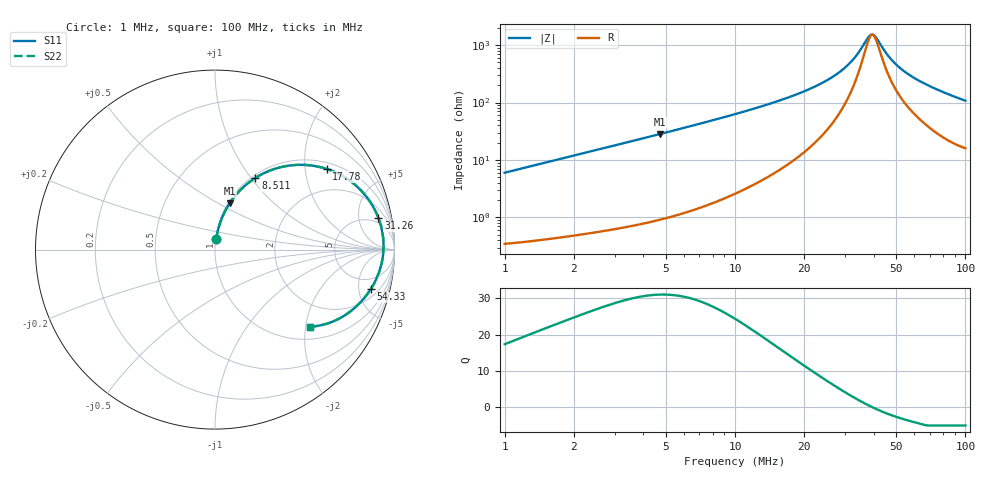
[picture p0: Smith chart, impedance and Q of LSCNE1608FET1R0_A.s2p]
! LSCNE1608FET1R0_A  S-PARAMETER MODEL  ( Standard Model )
! Model Generated by TAIYO YUDEN Corporation (http://www.ty-top.com)
! Version 1.0
! TAIYO YUDEN Control No. 160926
! Copyright(c) 2016 TAIYO YUDEN CO.,LTD. All Rights Reserved.
! Product Description (link to TY-COMPAS)
! https://ds.yuden.co.jp/TYCOMPAS/or/detail?pn=LSCNE1608FET1R0MA&u=M
! Products Name : Inductors
! Characteristics :
!  Inductance : 1.0 [uH] , SRF(min) : - [Hz] , DC Resistance(max) : 340 [mOhm]
!  Rated Current : Saturation  1.4 [A] (dL = 30 [%]), Temp Rise  0.8 [A] (dT = 40 [degC])
!  Case Size : 1.6 x 0.8 / 0.063 x 0.031 [mm/inch] , Thickness : 0.65 / 0.026 [mm/inch]
!  (Conditions: Temperature = 25 [degC] , DC Bias Current = 0 [A])
! External Node Assignments :
!  1  o---GGG---o  2
! GND o---------o GND
! Frequency Range : 1MHz  -  100MHz  [ 402 STEP ]
# MHz S RI R 50
! Freq[MHz].  S11 Real  S11 Imag  S21 Real  S21 Imag  S12 Real  S12 Imag  S22 Real  S22 Imag
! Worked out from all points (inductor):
!   401 points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, 1 MHz to 100 MHz, reference 50 ohm
!   read as one part in series: L = 952 nH near 1.023 MHz
!   highest Q = 31 at 4.732 MHz (marker M1), where L = 953 nH
!   self-resonance near 39.5 MHz
!   S11 on the Smith chart (normalised r, x): 1 MHz: 1.01, +0.12; 8.511 MHz: 1.04, +1.05; 17.78 MHz: 1.19, +2.61; 31.26 MHz: 3.61, +9.06; 54.33 MHz: 3.00, -6.67; 100 MHz: 1.32, -2.13
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1  0.007 0.0594  0.993 -0.0594  0.993 -0.0594  0.007 0.0594
1.62181  0.0135 0.0952  0.9865 -0.0952  0.9865 -0.0952  0.0135 0.0952
2.42661  0.0256 0.1401  0.9744 -0.1401  0.9744 -0.1401  0.0256 0.1401
3.467369  0.047 0.1956  0.953 -0.1956  0.953 -0.1956  0.047 0.1956
4.731513  0.0814 0.2578  0.9186 -0.2578  0.9186 -0.2578  0.0814 0.2578
6.456542  0.1407 0.3314  0.8593 -0.3314  0.8593 -0.3314  0.1407 0.3314
8.51138  0.2247 0.3992  0.7753 -0.3992  0.7753 -0.3992  0.2247 0.3992
12.73503  0.4148 0.4683  0.5852 -0.4683  0.5852 -0.4683  0.4148 0.4683
17.57924  0.6144 0.4519  0.3856 -0.4519  0.3856 -0.4519  0.6144 0.4519
17.78279  0.6218 0.4496  0.3782 -0.4496  0.3782 -0.4496  0.6218 0.4496
24.2661  0.8083 0.335  0.1917 -0.335  0.1917 -0.335  0.8083 0.335
31.26079  0.9108 0.1754  0.0892 -0.1754  0.0892 -0.1754  0.9108 0.1754
34.27678  0.9303 0.1077  0.0697 -0.1077  0.0697 -0.1077  0.9303 0.1077
38.01894  0.939 0.029  0.061 -0.029  0.061 -0.029  0.939 0.029
39.81072  0.9383 -0.00594  0.0617 0.00594  0.0617 0.00594  0.9383 -0.00594
41.20975  0.9359 -0.032  0.0641 0.032  0.0641 0.032  0.9359 -0.032
46.2381  0.9174 -0.1157  0.0826 0.1157  0.0826 0.1157  0.9174 -0.1157
50.69907  0.8919 -0.1777  0.1081 0.1777  0.1081 0.1777  0.8919 -0.1777
54.32503  0.8677 -0.2204  0.1323 0.2204  0.1323 0.2204  0.8677 -0.2204
67.6083  0.7682 -0.3333  0.2318 0.3333  0.2318 0.3333  0.7682 -0.3333
84.13951  0.641 -0.4069  0.359 0.4069  0.359 0.4069  0.641 -0.4069
100  0.5317 -0.4294  0.4683 0.4294  0.4683 0.4294  0.5317 -0.4294
